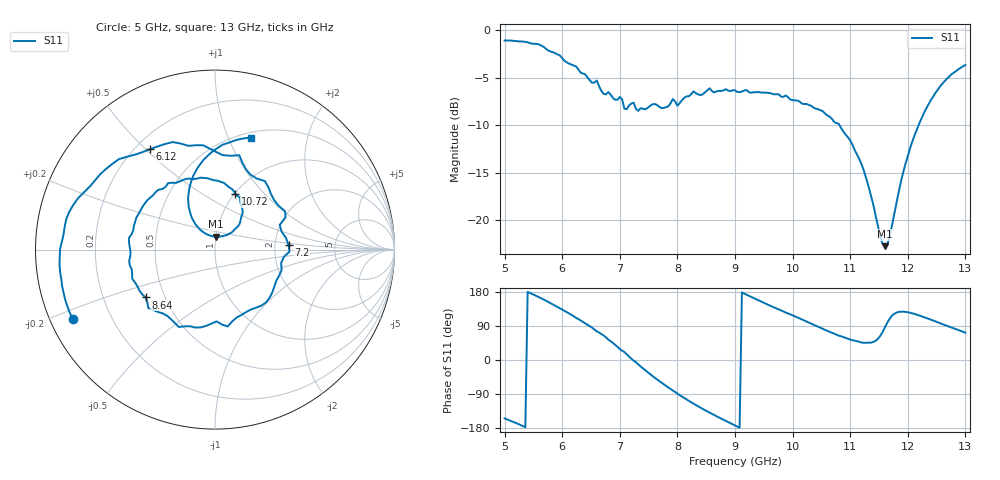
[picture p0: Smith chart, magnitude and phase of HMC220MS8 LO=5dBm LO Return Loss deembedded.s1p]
!Hittite Microwave Corporation
!12 Elizabeth Drive
!Chelmsford, MA 01824
!Tel: 978-250-3343
!Fax: 978-250-3373
!Device: HMC220MS8, 5-12 GHz, GaAS MMIC SMT Double-Balanced Mixer in 8-lead MSOP package
!Misc: LO power level=5dBm, Room
# MHZ S MA R 50
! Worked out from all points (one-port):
!   201 points, 5 GHz to 13 GHz, reference 50 ohm
!   lowest |S11| = -22.7 dB at 11.6 GHz (marker M1), VSWR 1.16, Z = 50.1 + j7.33 ohm
!   |S11| at or under -10 dB: 10.81 GHz to 12.19 GHz (1.374 GHz wide, 11.9 % of centre)
!   S11 on the Smith chart (normalised r, x): 5 GHz: 0.07, -0.23; 6.12 GHz: 0.26, +0.52; 7.2 GHz: 2.39, +0.14; 8.64 GHz: 0.39, -0.27; 10.72 GHz: 1.01, +0.70; 13 GHz: 0.56, +1.21
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5000  0.882 -154.0
5320  0.87 -174.5
5560  0.846 168.5
6000  0.712 133.4
6120  0.666 122.8
6240  0.644 111.5
6600  0.543 75.6
6720  0.462 64.7
7000  0.445 28.7
7080  0.386 21.0
7200  0.411 3.4
7600  0.409 -46.1
7920  0.434 -80.5
8000  0.4 -88.7
8280  0.476 -115.1
8640  0.47 -145.4
9000  0.482 -172.7
9560  0.468 146.6
10000  0.428 117.8
10320  0.4 96.1
10720  0.329 69.8
11000  0.263 53.9
11240  0.181 45.4
11600  0.073 85.0
11680  0.081 107.7
12000  0.218 126.1
12480  0.467 101.9
13000  0.655 72.2
